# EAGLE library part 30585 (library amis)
AMIS-30585 S-FSK PLC Modem Source: http://www.amis.com/pdf/amis_30585_ds.pdf
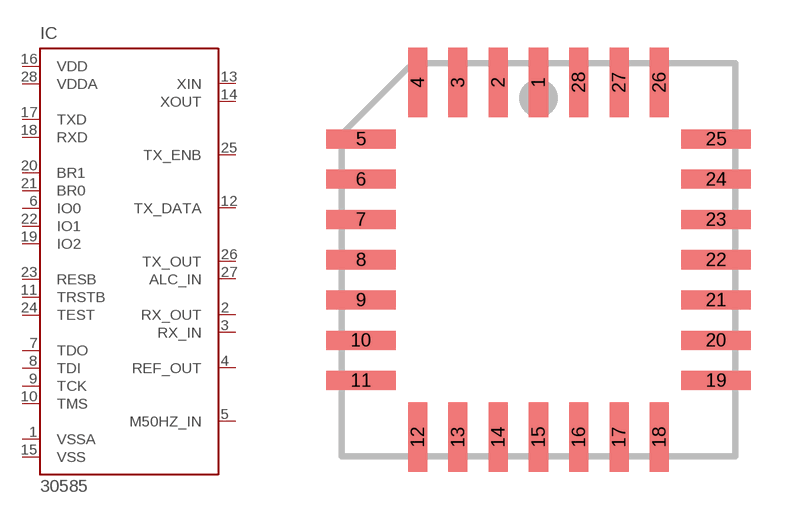
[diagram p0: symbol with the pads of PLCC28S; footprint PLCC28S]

Designator prefix IC

## 30585 (OC_FARNELL: unknown; OC_NEWARK: unknown)  [PLCC28S]
1  VSSA  in
2  RX_OUT  in
3  RX_IN  in
4  REF_OUT  in
5  M50HZ_IN  in
6  IO0  out
7  TDO  out
8  TDI  in
9  TCK  in
10  TMS  in
11  TRSTB  in
12  TX_DATA  out
13  XIN  in
14  XOUT  out
15  VSS  in
16  VDD  in
17  TXD  out
18  RXD  in
19  IO2  out
20  BR1  in
21  BR0  in
22  IO1  out
23  RESB  in
24  TEST  in
25  TX_ENB  out
26  TX_OUT  out
27  ALC_IN  in
28  VDDA  in

## Footprint PLCC28S (pad centres in mm)
PLASTIC LEADED CHIP CARRIER square
smd 0.6 x 2.2: 1 0,5.6; 2 -1.27,5.6; 3 -2.54,5.6; 4 -3.81,5.6; 12 -3.81,-5.6; 13 -2.54,-5.6; 14 -1.27,-5.6; 15 0,-5.6; 16 1.27,-5.6; 17 2.54,-5.6; 18 3.81,-5.6; 26 3.81,5.6; 27 2.54,5.6; 28 1.27,5.6
smd 2.2 x 0.6: 5 -5.6,3.81; 6 -5.6,2.54; 7 -5.6,1.27; 8 -5.6,0; 9 -5.6,-1.27; 10 -5.6,-2.54; 11 -5.6,-3.81; 19 5.6,-3.81; 20 5.6,-2.54; 21 5.6,-1.27; 22 5.6,0; 23 5.6,1.27; 24 5.6,2.54; 25 5.6,3.81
